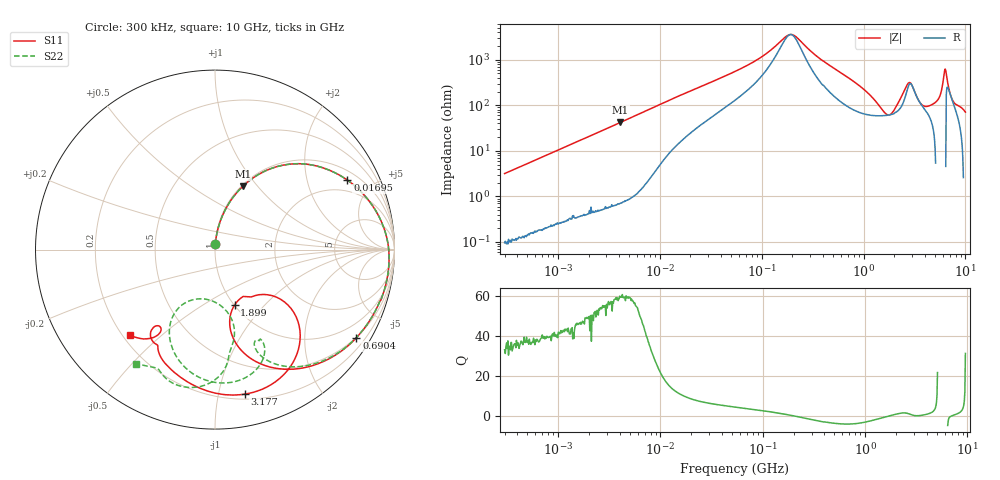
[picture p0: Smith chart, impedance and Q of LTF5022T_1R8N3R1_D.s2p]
! S-Parameter Data Generated by TDK Corporation
! Copyright(C) 2020 TDK Corporation.
! All Rights Reserved.
! TDK P/N: LTF5022T-1R8N3R1-D (Inductor)
! Property: L=1.8uH at 100kHz
! Size(LxWxT): 6.5x5x2.2mm
! Model Type: s2p (Touchstone File Format Version 1.0)
! Frequency: DC=Yes Start=0.3MHz Stop=10000MHz 802points Log-sweep
! Model Generated on Apr. 23, 2020
! Port Assignments:
!  1 ---@@@--- 2
! Applicable Conditions:
!  Temperature = 25 degC
!  DC Bias Current = 0 A
!  Small Signal Operation
! Terms and conditions regarding TDK Simulation Models
! (1)This simulation model is being provided solely for informational purposes. Please refer to the specifications of the products in terms of detailed characteristics of such products.
! (2)In no event shall TDK Corporation of any of its subsidiaries be liable for any loss or damage arising, directly or indirectly,
!  From any information contained in this simulation model, including, but not limited to loss or damages arising from any inaccuracies, omissions or errors in connection with such information.
! (3)Any and all copyrights on this simulation model are owned by TDK Corporation.
!  Duplication or redistribution of this simulation model without prior written permission from TDK Corporation is prohibited.
! (4)This simulation model is subject to any modification or change without any prior notice.
! (5)Neither TDK Corporation nor any of its subsidiaries shall make any warranty, express or implied,
!  Including but not limited to the correctness, implied warranties of merchantability and fitness for a particular purpose with respect to this simulation models.
! (6)The use of this simulation model shall be deemed to have consented to the terms and conditions hereof.
# Hz S MA R 50
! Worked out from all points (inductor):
!   801 points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, 300 kHz to 10 GHz, reference 50 ohm
!   read as one part in series: L = 1.68 uH near 318.3 kHz
!   highest Q = 59.6 at 4.116 MHz (marker M1), where L = 1.63 uH
!   self-resonance near 192.2 MHz
!   S11 on the Smith chart (normalised r, x): 300 kHz: 1.00, +0.06; 16.95 MHz: 1.40, +3.54; 690.4 MHz: 0.48, -3.43; 1.899 GHz: 1.01, -0.69; 3.177 GHz: 0.24, -1.20; 10 GHz: 0.23, -0.40
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300000  0.03196 86.6  0.9987 -1.8  0.9984 -1.8  0.03166 86.3
1713600  0.1724 78.8  0.9813 -10.0  0.9813 -10.0  0.1725 78.8
4115543  0.3854 66.3  0.9164 -22.8  0.9163 -22.8  0.3853 66.3
9671944  0.6953 43.2  0.6891 -44.3  0.6891 -44.3  0.6953 43.2
1.694973e7  0.8333 27.7  0.4745 -56.5  0.4745 -56.5  0.8333 27.7
5.477226e7  0.946 8.0  0.1714 -68.5  0.1714 -68.5  0.946 8.0
1.878293e8  0.9726 -5.3  0.02732 -10.8  0.02733 -10.8  0.9726 -5.2
3.126428e8  0.9708 -12.6  0.06601 53.5  0.06602 53.5  0.9709 -12.3
6.904357e8  0.9282 -32.0  0.2069 46.0  0.2069 45.9  0.9303 -31.0
1.228555e9  0.7618 -60.9  0.4043 11.7  0.404 11.6  0.785 -56.3
1.767019e9  0.4066 -78.4  0.5273 -35.2  0.5259 -35.4  0.5697 -67.4
1.898818e9  0.3269 -70.4  0.5237 -48.4  0.522 -48.6  0.5547 -65.5
2.203374e9  0.4338 -37.7  0.4339 -78.4  0.4307 -78.9  0.6257 -63.7
2.507534e9  0.6741 -45.2  0.2641 -99.5  0.2586 -100.2  0.7326 -76.3
2.840323e9  0.803 -63.3  0.1454 -85.1  0.1379 -83.9  0.728 -94.3
3.177248e9  0.8221 -78.4  0.1764 -64.8  0.1737 -61.9  0.6426 -108.8
4.107799e9  0.7468 -103.0  0.2702 -96.0  0.2759 -93.5  0.3489 -120.1
4.924213e9  0.6884 -114.3  0.251 -139.0  0.2655 -136.2  0.3363 -80.7
5.607117e9  0.6366 -119.9  0.1652 172.3  0.1889 175.3  0.5252 -78.9
6.41458e9  0.6188 -123.9  0.04456 19.1  0.05277 42.0  0.6678 -85.4
7.652089e9  0.5313 -127.0  0.1801 -100.6  0.1812 -97.5  0.7749 -109.4
1e10  0.6702 -134.6  0.2051 164.0  0.2093 162.9  0.7749 -124.7
